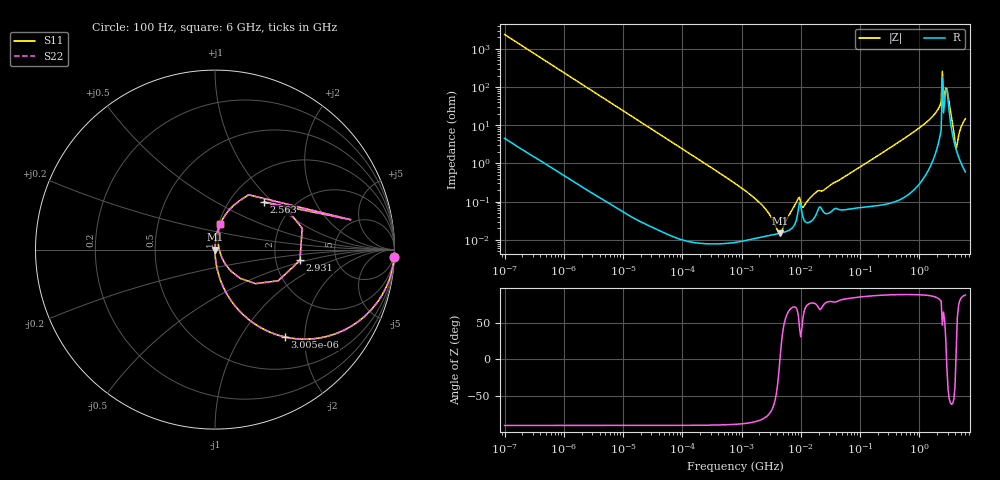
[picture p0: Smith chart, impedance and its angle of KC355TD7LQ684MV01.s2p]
!Murata Part Number: KC355TD7LQ684MV01
!These Parameters are Measured in Series Mode Connection
!Data Generated on Jun 19, 2026
!  o--ll--o
!Port1  Port2
!  o------o
!Operation Temp=25[degC], DC Bias Voltage=0[V]
!Freq. Start=100[Hz] Stop=6[GHz] 401[Steps]
# Hz S RI R 50
!Freq.(Hz) S11(Real) S11(Imag) S21(Real) S21(Imag) S12(Real) S12(Imag) S22(Real) S22(Imag)
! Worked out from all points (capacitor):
!   401 points, 100 Hz to 6 GHz, reference 50 ohm
!   read as one part in series: C = 664 nF near 109 Hz
!   lowest |Z| = 14.9 mohm at 4.441 MHz (marker M1)
!   series resonance near 4.442 MHz, so ESL is about 1.9 nH
!   S11 on the Smith chart (normalised r, x): 100 Hz: 1, -48; 3.005 kHz: 1.00, -1.60; 2.563 GHz: 1.42, +0.88; 2.931 GHz: 2.75, -0.43; 6 GHz: 1.01, +0.30
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100  0.9982 -0.0417  0.00182 0.0417  0.00182 0.0417  0.9982 -0.0417
686  0.924 -0.264  0.076 0.264  0.076 0.264  0.924 -0.264
2008  0.5885 -0.4911  0.4115 0.4911  0.4115 0.4911  0.5885 -0.4911
3005  0.3904 -0.4868  0.6096 0.4868  0.6096 0.4868  0.3904 -0.4868
8047  0.0826 -0.2742  0.9174 0.2742  0.9174 0.2742  0.0826 -0.2742
40335  0.00374 -0.0596  0.9963 0.0596  0.9963 0.0596  0.00374 -0.0596
774597  9.45e-05 -0.003  0.9999 0.003  0.9999 0.003  9.45e-05 -0.003
2268635  0.000121 -0.000771  0.9999 0.000771  0.9999 0.000771  0.000121 -0.000771
4440638  0.000149 -4e-07  0.9999 4e-07  0.9999 4e-07  0.000149 -4e-07
8692127  0.000413 0.000988  0.9996 -0.000988  0.9996 -0.000988  0.000413 0.000988
1.137099e7  0.000326 0.000711  0.9997 -0.000711  0.9997 -0.000711  0.000326 0.000711
1.555665e7  0.000325 0.00138  0.9997 -0.00138  0.9997 -0.00138  0.000325 0.00138
3.124326e8  0.00153 0.025  0.9985 -0.025  0.9985 -0.025  0.00153 0.025
1.791126e9  0.0485 0.1795  0.9515 -0.1795  0.9515 -0.1795  0.0485 0.1795
2.142435e9  0.1051 0.247  0.8949 -0.247  0.8949 -0.247  0.1051 0.247
2.562649e9  0.2705 0.2651  0.7295 -0.2651  0.7295 -0.2651  0.2705 0.2651
2.679998e9  0.3893 0.2398  0.6107 -0.2398  0.6107 -0.2398  0.3893 0.2398
2.931063e9  0.4735 -0.06  0.5265 0.06  0.5265 0.06  0.4735 -0.06
3.352442e9  0.1405 -0.1601  0.8595 0.1601  0.8595 0.1601  0.1405 -0.1601
3.8344e9  0.0401 -0.0492  0.9599 0.0492  0.9599 0.0492  0.0401 -0.0492
4.193612e9  0.0225 0.0048  0.9775 -0.0048  0.9775 -0.0048  0.0225 0.0048
6e9  0.0272 0.1438  0.9728 -0.1438  0.9728 -0.1438  0.0272 0.1438
